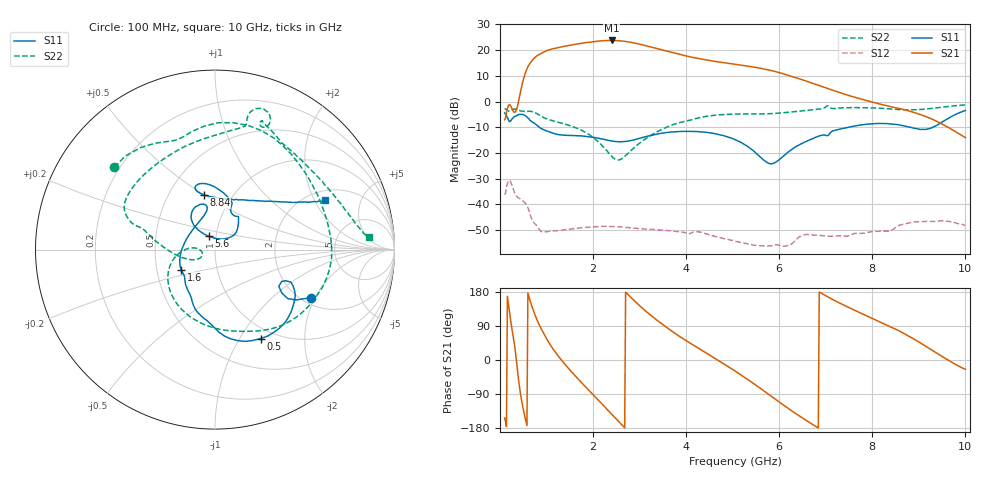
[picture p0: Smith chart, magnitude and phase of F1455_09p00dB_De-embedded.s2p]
! Integrated Device Technology
! Corporate Headquarters
! 6024 Silver Creek Valley Road
! San Jose, CA 95138  USA
! Phone:  1-408-284-8200
! Toll Free:  1-800-223-1366
! Webpage:  http://www.idt.com/
! Timing and RF Division
! 515 Groton Road, Suite 102
! Westford, MA 01886-6024
! Device:  F1455
! Description: 6-bit 0.5 dB Transmit Variable Gain Amplifier
! Frequency:  1400.0 -  2300.00 MHz
! Package:  6x6 mm Thin QFN Plastic Package: 28 pin
! State:  18
! Atten State:  9.0 dB
! Voltage:  +5.00 Volts
! Current:  217.693 mA
! Data:  The device was measured on a the F1455 evaluation board which has
!  individual transmission lines to the RF pins.  Data was collected
!  using a calibrated network analyzer.  The evaluation board was
!  de-embedded using a TRL calibration technique.
!  The reference plane is the edge of the package pin.
!  Pin  1 = CSb
!  Pin  2 = DATA
!  Pin  3 = CLK
!  Pin  4 = RSET
!  Pin  5 = GND
!  Pin  6 = RFIN  = Port 1
!  Pin  7 = GND
!  Pin  8 = NC
!  Pin  9 = NC
!  Pin 10 = NC
!  Pin 11 = NC
!  Pin 12 = NC
!  Pin 13 = NC
!  Pin 14 = /STBY
!  Pin 15 = GND
!  Pin 16 = RFOUT  = Port 2
!  Pin 17 = GND
!  Pin 18 = NC
!  Pin 19 = NC
!  Pin 20 = NC
!  Pin 21 = GND
!  Pin 22 = NC
!  Pin 23 = GND
!  Pin 24 = NC
!  Pin 25 = NC
!  Pin 26 = NC
!  Pin 27 = GND
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# GHz S dB R 50
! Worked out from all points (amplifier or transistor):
!   496 points, 100 MHz to 10 GHz, reference 50 ohm
!   highest |S21| = 23.8 dB at 2.4 GHz (marker M1)
!   |S21| within 3 dB of that: 1.194 GHz to 3.344 GHz (2.15 GHz wide, 94.8 % of centre)
!   unconditionally stable (mu >= 1): start of sweep to end of sweep
!   at 1.74 GHz: K = 9.19, MAG = 23.2 dB, |S12| = -49.1 dB
!   at 5.06 GHz: K = 31.78, MAG = 16.4 dB, |S12| = -54.3 dB
!   at 10 GHz: K = 89.11, MAG = -5.5 dB, |S12| = -48.1 dB
!   S11 on the Smith chart (normalised r, x): 100 MHz: 2.22, -1.88; 500 MHz: 0.86, -1.24; 1.6 GHz: 0.67, -0.16; 5.6 GHz: 0.92, +0.14; 8.84 GHz: 0.74, +0.50; 10 GHz: 2.44, +2.44
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0.1  -4.42 -26.7  -7.02 -152.9  -36.13 44.7  -2.80 140.7
0.38  -5.23 -39.1  -1.49 -31.1  -37.17 -111.5  -3.22 56.4
0.5  -5.08 -62.8  8.44 -129.7  -38.74 -149.3  -3.77 27.8
0.68  -7.75 -94.3  15.74 143.9  -45.60 149.7  -3.85 -14.4
0.82  -9.58 -111.3  18.09 99.0  -49.06 132.3  -4.92 -47.1
0.96  -11.08 -121.3  19.49 65.6  -50.70 123.9  -6.39 -71.8
1.26  -12.83 -138.1  21.05 9.3  -50.11 89.1  -8.06 -111.9
1.6  -13.20 -148.9  22.23 -39.6  -49.37 57.9  -9.95 -145.2
1.76  -13.34 -154.6  22.69 -60.7  -49.00 45.8  -11.20 -157.9
2.08  -14.11 -169.9  23.47 -101.6  -48.59 23.9  -15.08 -178.5
2.4  -15.30 164.2  23.78 -142.9  -48.55 4.3  -21.28 179.9
2.58  -15.63 145.6  23.63 -166.0  -48.75 -5.8  -22.56 -159.6
2.76  -15.34 127.5  23.23 171.5  -48.99 -14.5  -19.97 -150.5
3.06  -13.97 107.5  22.09 136.8  -49.43 -27.4  -15.34 -162.7
3.4  -12.53 100.6  20.51 102.5  -49.87 -40.1  -11.53 -179.9
4.1  -11.58 110.9  17.34 43.5  -51.08 -61.0  -7.14 163.5
5.06  -14.85 130.6  14.50 -29.7  -54.32 -98.9  -4.84 148.5
5.6  -21.64 115.1  12.95 -75.2  -56.04 -103.5  -4.79 127.2
6.7  -14.53 46.7  7.23 -168.9  -51.80 -138.0  -3.20 78.4
8.36  -8.61 106.7  -1.85 89.3  -50.34 167.2  -2.82 62.5
8.84  -10.11 101.7  -3.92 58.8  -47.03 150.0  -3.19 44.2
10  -3.46 24.1  -14.02 -24.3  -48.06 78.8  -1.29 4.7
